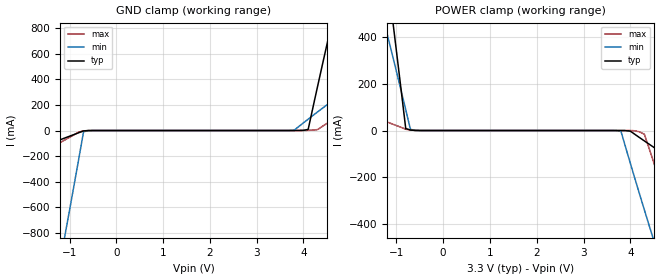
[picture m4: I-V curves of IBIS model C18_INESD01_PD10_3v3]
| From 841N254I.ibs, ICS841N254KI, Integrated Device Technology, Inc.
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[Model] C18_INESD01_PD10_3v3
Model_type   Input
Polarity   Non-Inverting
Vinl = 0.8V
Vinh = 2.0V
|   typ   min   max
C_comp   2pF   1.5pF   2.5pF
|   typ   min   max
[Voltage range]   3.3V   3.135V   3.465V
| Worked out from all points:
|   GND clamp passes 1 mA (typ) near -0.62 V on its own axis
|   POWER clamp passes 1 mA (typ) near -0.63 V on its own axis
[GND_clamp]
|Voltage   I (typ)   I (min)   I (max)
-3.3V     -328.3mA   -4.771A    -474.7mA
-2.2V     -200.9mA   -2.908A    -285.4mA
-1.1V     -58.5mA    -826.1mA   -73.83mA
-1V       -44.76mA   -625.2mA   -53.42mA
-700mV    -2.701mA   -10.28mA   -3.627mA
3.8V      93.26uA    2.307mA    40.42uA
4.1V      8.306mA    89.1mA     1.129mA
4.3V      343.2mA    145.5mA    7.196mA
4.5V      671.5mA    200.8mA    56.11mA
4.6V      833.1mA    228.1mA    80.2mA
5.6V      2.363A     485.9mA    308.2mA
6.6V      3.748A     719mA      514.5mA
[Power_clamp]
|Voltage   I (typ)   I (min)   I (max)
-3.3V     3.748A     1.938A     181.6mA
-1.3V     833.1mA    497mA      44.51mA
-1.1V     508.2mA    336.4mA    29.22mA
-1V       343.2mA    254.9mA    21.46mA
-800mV    8.306mA    89.34mA    5.708mA
-700mV    2.015mA    5.311mA    2.514mA
-600mV    528.8uA    598.8uA    639.8uA
3.8V      -50.69uA   -3.819mA   -3.656uA
4.2V      -30.88mA   -275.3mA   -5.932mA
4.5V      -72.1mA    -471.9mA   -137.5mA
5V        -138.1mA   -786.7mA   -430.2mA
6.6V      -328.3mA   -1.694A    -1.274A
